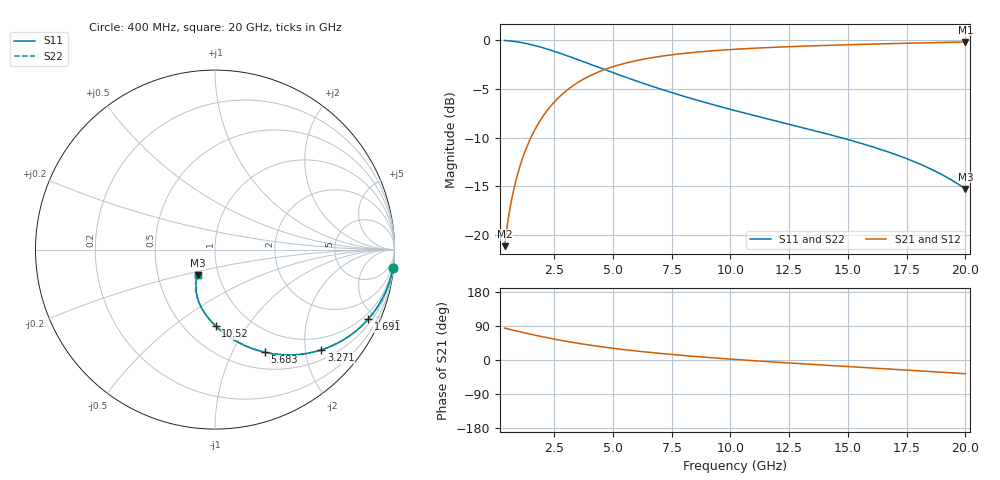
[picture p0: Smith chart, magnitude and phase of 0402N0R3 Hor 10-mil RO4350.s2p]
# GHz S MA R 50
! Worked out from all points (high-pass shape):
!   1960 points, 400 MHz to 20 GHz, reference 50 ohm
!   highest |S21| = -0.19 dB at 20 GHz (marker M1); lowest = -21.1 dB at 400 MHz (marker M2)
!   |S21| within 3 dB of the highest: 4.47 GHz to end of sweep
!   lowest |S11| = -15.3 dB at 20 GHz (marker M3), VSWR 1.42, Z = 39.6 - j11.6 ohm
!   |S11| at or under -10 dB: 14.7 GHz to end of sweep
!   |S22| runs from -15.3 to 0.0 dB; largest |S21 - S12| = 0
!   S11 on the Smith chart (normalised r, x): 400 MHz: 1, -19; 1.691 GHz: 0.71, -4.51; 3.271 GHz: 0.70, -2.34; 5.683 GHz: 0.70, -1.35; 10.52 GHz: 0.70, -0.72; 20 GHz: 0.79, -0.23
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0.4  0.9961 -6.0  0.08776 84.0  0.08776 84.0  0.9961 -6.0
0.4600306  0.9949 -6.9  0.1008 83.1  0.1008 83.1  0.9949 -6.9
0.6801429  0.9889 -10.2  0.1481 79.8  0.1481 79.8  0.9889 -10.2
0.9402757  0.9792 -14.0  0.2026 76.0  0.2026 76.0  0.9792 -14.0
1.280449  0.9625 -18.8  0.2709 71.2  0.2709 71.2  0.9625 -18.8
1.690658  0.9374 -24.4  0.3479 65.5  0.3479 65.5  0.9374 -24.4
2.020827  0.9141 -28.8  0.4049 61.2  0.4049 61.2  0.9141 -28.8
2.391016  0.8858 -33.4  0.4633 56.6  0.4633 56.6  0.8858 -33.4
2.821235  0.8512 -38.4  0.5239 51.6  0.5239 51.6  0.8512 -38.4
3.271465  0.8144 -43.3  0.5794 46.7  0.5794 46.7  0.8144 -43.3
3.671669  0.7819 -47.3  0.6223 42.6  0.6223 42.6  0.7819 -47.3
4.67218  0.7052 -56.3  0.7077 33.6  0.7077 33.6  0.7052 -56.3
5.682695  0.637 -64.0  0.7693 25.9  0.7693 25.9  0.637 -64.0
6.943338  0.5657 -72.0  0.8227 17.8  0.8227 17.8  0.5657 -72.0
8.464114  0.497 -80.2  0.8655 9.6  0.8655 9.6  0.497 -80.2
10.205  0.4352 -88.2  0.8977 1.5  0.8977 1.5  0.4352 -88.2
10.51516  0.4255 -89.5  0.9022 0.2  0.9022 0.2  0.4255 -89.5
11.93589  0.3851 -95.3  0.9198 -5.6  0.9198 -5.6  0.3851 -95.3
13.46667  0.3461 -101.0  0.9346 -11.5  0.9346 -11.5  0.3461 -101.0
16.73834  0.2665 -112.8  0.959 -23.6  0.959 -23.6  0.2665 -112.8
18.50924  0.2189 -119.0  0.9701 -30.3  0.9701 -30.3  0.2189 -119.0
20  0.1726 -124.3  0.9784 -36.2  0.9784 -36.2  0.1726 -124.3
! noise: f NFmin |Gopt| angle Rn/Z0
0.4  0.002014  0.9167  5.222  0.005327
2.571  0.004677  0.6923  14.19  0.002918
4.752  0.007201  0.6213  18.34  0.003464
6.933  0.009616  0.5873  22.57  0.004106
9.104  0.01203  0.5697  26.87  0.004799
11.29  0.01454  0.5623  31.2  0.005578
13.47  0.01725  0.5625  35.45  0.006487
15.64  0.02023  0.569  39.58  0.00758
17.82  0.02364  0.5812  43.62  0.008955
20  0.02762  0.5986  47.53  0.01074
